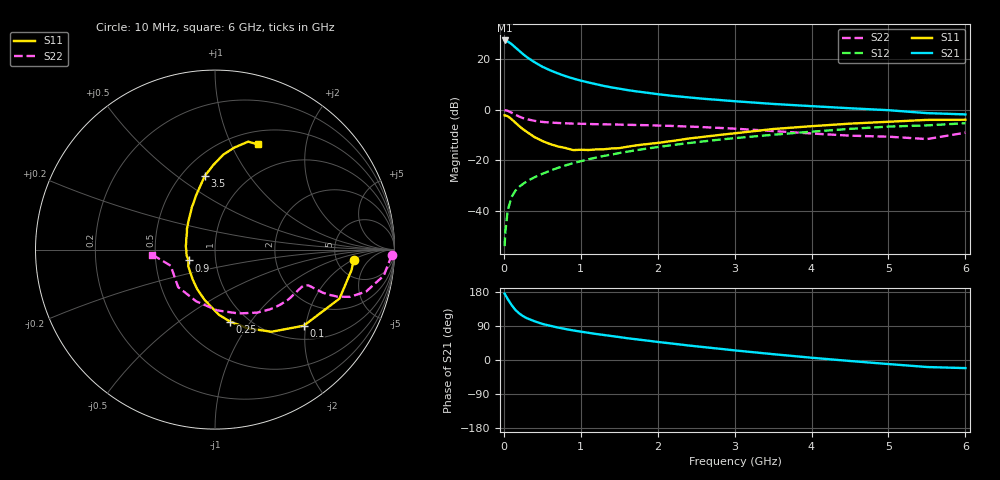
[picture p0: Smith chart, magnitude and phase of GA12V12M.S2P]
! Infineon Technologies  Discrete & RF Semiconductors
! BF775
! Si NPN RF Bipolar Junction Transistor in SOT23
! VCE = 12 V  IC = 12 mA
! Common Emitter S-Parameters:  May  1996
# GHz  S  MA  R  50
!  f  S11  S21  S12  S22
! GHz  MAG  ANG  MAG  ANG  MAG  ANG  MAG  ANG
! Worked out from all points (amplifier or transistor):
!   36 points, 10 MHz to 6 GHz, reference 50 ohm
!   highest |S21| = 27.4 dB at 10 MHz (marker M1)
!   |S21| within 3 dB of that: start of sweep to 158.4 MHz
!   unconditionally stable (mu >= 1): 603.5 MHz to 2.685 GHz
!   at 250 MHz: K = 0.69, MSG = 25.7 dB, |S12| = -29.3 dB
!   at 1.4 GHz: K = 1.09, MAG = 11.5 dB, |S12| = -17.7 dB
!   at 6 GHz: K = 0.87, MSG = 1.7 dB, |S12| = -5.3 dB
!   S11 on the Smith chart (normalised r, x): 10 MHz: 7.22, -2.14; 100 MHz: 1.32, -1.95; 250 MHz: 0.83, -0.80; 900 MHz: 0.74, -0.09; 3.5 GHz: 0.64, +0.64; 6 GHz: 0.65, +1.28
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0.01  0.7745 -4.4  23.45 175.2  0.002 86.0  0.9851 -1.7
0.02  0.7691 -8.6  22.97 171.5  0.0039 79.7  0.9752 -3.6
0.05  0.7453 -21.5  22.41 161.0  0.0101 77.6  0.9511 -8.8
0.1  0.6515 -40.6  19.93 145.3  0.0187 71.3  0.874 -15.5
0.15  0.5554 -55.5  17.02 132.2  0.025 66.6  0.7967 -19.3
0.2  0.4736 -67.6  14.65 122.9  0.0299 65.4  0.732 -21.0
0.25  0.4103 -78.1  12.57 115.7  0.0342 64.0  0.683 -21.6
0.3  0.3637 -86.6  10.96 110.3  0.0385 63.8  0.6492 -21.8
0.4  0.2865 -101.6  8.695 102.1  0.0463 64.6  0.6027 -21.4
0.5  0.241 -114.4  7.1 95.3  0.0539 65.6  0.574 -21.1
0.6  0.2096 -125.8  6.041 90.4  0.0622 66.4  0.5582 -21.0
0.7  0.188 -137.1  5.251 85.8  0.0706 66.8  0.5473 -21.3
0.9  0.159 -157.6  4.148 78.1  0.0877 67.1  0.5317 -22.3
1.1  0.1595 -177.5  3.462 71.8  0.1047 67.1  0.5224 -24.3
1.3  0.1651 166.6  2.956 66.0  0.1219 66.1  0.5146 -26.4
1.6  0.1848 147.7  2.456 57.6  0.1475 64.3  0.5029 -30.4
2.2  0.2418 124.7  1.874 43.1  0.2007 59.9  0.4769 -39.8
2.8  0.3168 109.7  1.559 29.8  0.2556 54.5  0.4367 -51.5
3.5  0.415 97.8  1.302 15.4  0.3199 47.0  0.3787 -69.9
4.5  0.5311 85.0  1.069 -2.6  0.4179 35.2  0.3067 -109.8
5.5  0.6292 72.9  0.857 -18.5  0.4896 19.9  0.2628 -160.1
6  0.6335 67.6  0.808 -21.4  0.5415 15.8  0.3516 -175.5
